FUNCTION FC 96 : VOID
TITLE =COMANDO VELOCITA' MOTORE PRESSA
AUTHOR : Esposito
FAMILY : EGAL_srl
NAME : CO_CU_BR
VERSION : 0.1


VAR_TEMP
  COUNTER_Z11 : INT ;
END_VAR
BEGIN
NETWORK
TITLE =CONTROL SPEED FOR CLUCTH/BRAKE
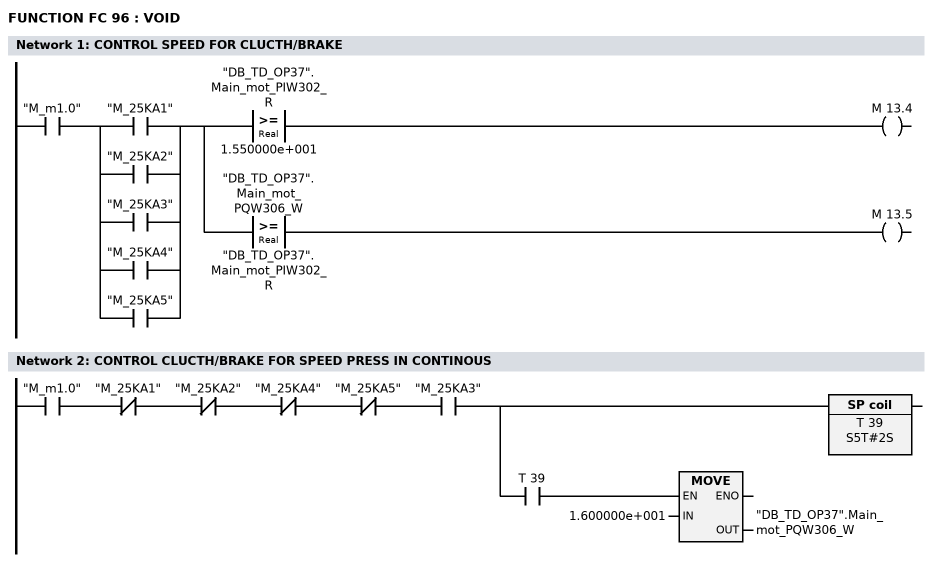
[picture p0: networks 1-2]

      U     "M_m1.0";
      U(    ;
      O     "M_25KA1";
      O     "M_25KA2";
      O     "M_25KA3";
      O     "M_25KA4";
      O     "M_25KA5";
      )     ;
      =     L      2.0;
      U     L      2.0;
      U(    ;
      L     "DB_TD_OP37".Main_mot_PIW302_R;
      L     1.550000e+001;
      >=R   ;
      )     ;
      =     M     13.4;
      U     L      2.0;
      U(    ;
      L     "DB_TD_OP37".Main_mot_PQW306_W;
      L     "DB_TD_OP37".Main_mot_PIW302_R;
      >=R   ;
      )     ;
      =     M     13.5;
NETWORK
TITLE =CONTROL CLUCTH/BRAKE FOR SPEED PRESS IN CONTINOUS

      U     "M_m1.0";
      UN    "M_25KA1";
      UN    "M_25KA2";
      UN    "M_25KA4";
      UN    "M_25KA5";
      U     "M_25KA3";
      =     L      2.0;
      U     L      2.0;
      BLD   102;
      L     S5T#2S;
      SI    T     39;
      U     L      2.0;
      U     T     39;
      SPBNB _001;
      L     1.600000e+001;
      T     "DB_TD_OP37".Main_mot_PQW306_W;
_001: NOP   0;
NETWORK
TITLE =LOAD VALUE AFTER CLUTCH/BRAKE

      U     "M_m1.0";
      U     "M_25KA3";
      =     L      2.0;
      U     L      2.0;
      U     M     13.4;
      U     M     13.5;
      U     "M_108KA1_2";
      U     "M_37KA1";
      FP    M     13.6;
      ZV    Z     11;
      NOP   0;
      U     M     13.7;
      L     C#3;
      S     Z     11;
      U     M     14.5;
      R     Z     11;
      NOP   0;
      NOP   0;
      NOP   0;
      U     L      2.0;
      BLD   102;
      =     M     13.7;
      U(    ;
      U     L      2.0;
      SPBNB _002;
      L     Z     11;
      T     #COUNTER_Z11;
      SET   ;
      SAVE  ;
      CLR   ;
_002: U     BIE;
      )     ;
      U(    ;
      L     #COUNTER_Z11;
      L     3;
      ==I   ;
      )     ;
      =     M     14.5;
NETWORK
TITLE =INCREASE VALUE IN CONTINUOUS
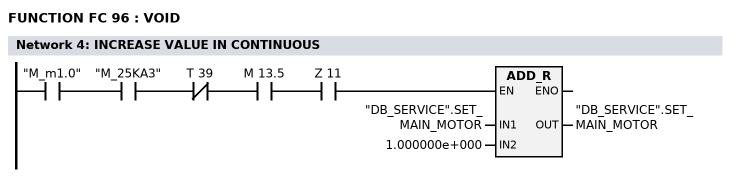
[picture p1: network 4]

      U     "M_m1.0";
      U     "M_25KA3";
      UN    T     39;
      U     M     13.5;
      U     Z     11;
      SPBNB _003;
      L     "DB_SERVICE".SET_MAIN_MOTOR;
      L     1.000000e+000;
      +R    ;
      T     "DB_SERVICE".SET_MAIN_MOTOR;
_003: NOP   0;
END_FUNCTION

